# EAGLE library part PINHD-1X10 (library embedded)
PIN HEADER
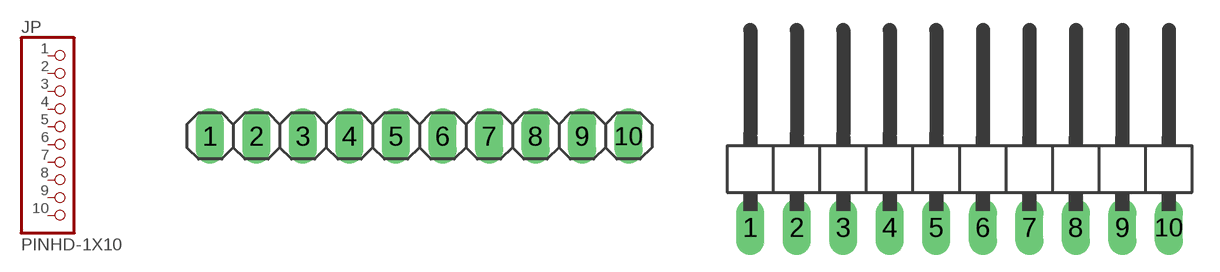
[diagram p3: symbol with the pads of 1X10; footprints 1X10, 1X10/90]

Designator prefix JP

## PINHD-1X10 (ANGLE: Straight; PACKAGE: Pin Header; PITCH: 2.54mm; POS: 10; ROWS: 10)  [1X10]
1  1  pas
2  2  pas
3  3  pas
4  4  pas
5  5  pas
6  6  pas
7  7  pas
8  8  pas
9  9  pas
10  10  pas

## PINHD-1X10/90 (ANGLE: 90; PACKAGE: Pin Header; PITCH: 2.54mm; POS: 10; ROWS: 1)  [1X10/90]
Pads as for 1X10

## Footprint 1X10 (pad centres in mm)
PIN HEADER
drill 1.016 long: 1 -11.43,0; 2 -8.89,0; 3 -6.35,0; 4 -3.81,0; 5 -1.27,0; 6 1.27,0; 7 3.81,0; 8 6.35,0; 9 8.89,0; 10 11.43,0

## Footprint 1X10/90 (pad centres in mm)
PIN HEADER
drill 1.016 long: 1 -11.43,-3.81; 2 -8.89,-3.81; 3 -6.35,-3.81; 4 -3.81,-3.81; 5 -1.27,-3.81; 6 1.27,-3.81; 7 3.81,-3.81; 8 6.35,-3.81; 9 8.89,-3.81; 10 11.43,-3.81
